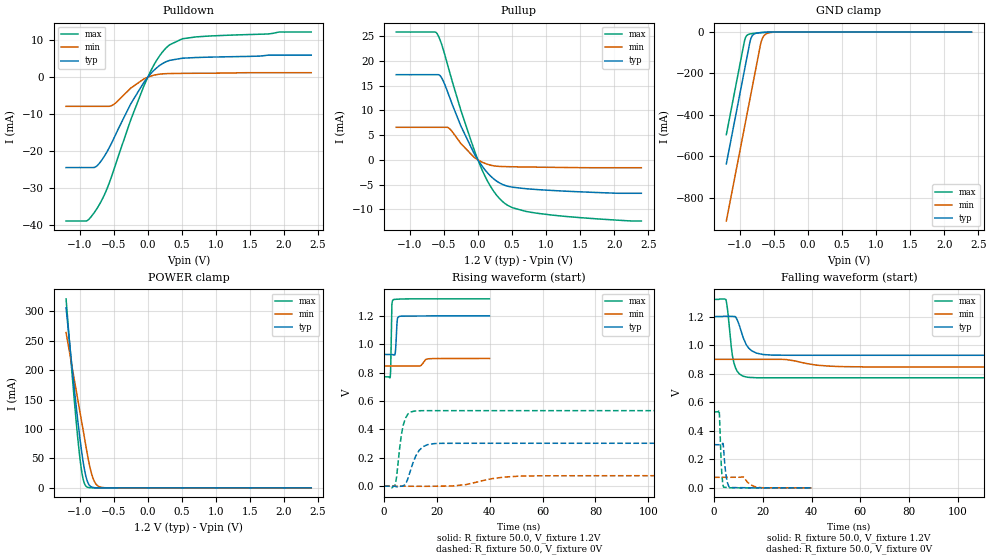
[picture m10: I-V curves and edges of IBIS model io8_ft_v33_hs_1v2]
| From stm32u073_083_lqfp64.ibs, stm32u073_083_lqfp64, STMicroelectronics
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[Model]   io8_ft_v33_hs_1v2
Model_type I/O
Polarity   Non-Inverting
Enable   Active-Low
| CAP_THRESHOLD on pad IOFT is "UDTCAPC" :
| Rising=30.0% of vddiom   Falling=70.0% of vddiom
| C_comp min and max val. don't necessarily correlate with the min and max pvt
| but are the smallest and greatest pad capacitance found.
| var   typ   min   max
C_comp   1.89804pF  1.82360pF  1.89870pF
|C_comp_pullup   1.10155pF  1.05685pF  1.08560pF
|C_comp_pulldown   796.48500fF  766.74501fF  813.10001fF
Vinl = 270.0mV
Vinh = 924.0mV
Vmeas = 600.0mV   | Reference voltage for timing measurements
Cref  = 50.0pF   | Timing specification test load capacitance value
Rref  = 100.0MOhm   | Timing specification test load resistance value
Vref  = 600.0mV   | Timing specification test load voltage
[Model Spec]
| TIME_THRESHOLD on pin ZIV33M is "CMOS" :
| Rising=50.0% of vddiom   Falling=50.0% of vddiom
Vinl 458.70000mV 364.70000mV 499.70000mV
Vinh 728.30000mV 548.30000mV 792.30000mV
| variable   typ   min   max
[Temperature Range] 25.0 140.0 -40.0
| variable   typ   min   max
[Voltage Range] 1.2V 900.0mV 1.32V
| variable   typ   min   max
[POWER Clamp Reference] 1.2V 900.0mV 1.32V
| variable   typ   min   max
[GND Clamp Reference] 0V 0V 0V
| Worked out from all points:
|   slope of the pulldown table from 0 to 0.18 V, typ, clamps not added: 55.6 ohm
|   slope of the pullup table from 0 to 0.18 V, typ, clamps not added: 56.3 ohm
|   GND clamp passes 1 mA (typ) near -0.61 V on its own axis
|   POWER clamp passes 1 mA (typ) near -0.81 V on its own axis
|   rising waveform, R_fixture 50.0, V_fixture 1.2V: 20-80 % time 435ps typ, 1.27ns min, 277ps max; typ from 0.928 V to 1.2 V
|   falling waveform, R_fixture 50.0, V_fixture 1.2V: 20-80 % time 3.79ns typ, 10.5ns min, 2.27ns max; typ from 1.2 V to 0.928 V
|   rising waveform, R_fixture 50.0, V_fixture 0V: 20-80 % time 3.76ns typ, 11.5ns min, 2.21ns max; typ from 0 V to 0.302 V
|   falling waveform, R_fixture 50.0, V_fixture 0V: 20-80 % time 1.14ns typ, 2.92ns min, 784ps max; typ from 0.302 V to 0 V
[POWER Clamp]
-1.2V     306.2mA    263.9mA    321.2mA
-1.09V    180mA      191mA      163.4mA
-1.05V    136.9mA    164.5mA    110.9mA
-1.01V    96.55mA    138mA      64.02mA
-960mV    52.29mA    104.9mA    20.68mA
-930mV    31.08mA    85.01mA    7.282mA
-900mV    15.67mA    65.13mA    2.025mA
-850mV    3.417mA    35.2mA     196.2uA
-800mV    570.2uA    14.97mA    18.13uA
-750mV    88.98uA    4.952mA    1.667uA
-680mV    6.495uA    823.9uA    58.96nA
2.4V      0A         0A         0A
[GND Clamp]
-1.2V     -636.9mA   -913.2mA   -495.8mA
-940mV    -194.9mA   -471.2mA   -53.78mA
-920mV    -160.9mA   -437.2mA   -28.06mA
-890mV    -109.9mA   -386.2mA   -14.28mA
-850mV    -43.09mA   -318.2mA   -9.18mA
-820mV    -18.33mA   -267.2mA   -7.516mA
-780mV    -7.695mA   -199.2mA   -5.87mA
-690mV    -2.548mA   -49.42mA   -2.9mA
-660mV    -1.868mA   -24.06mA   -2.112mA
-630mV    -1.326mA   -12.18mA   -1.447mA
-430mV    -19.32uA   -177.8uA   -8.091uA
2.4V      298.5pA    77.04nA    207.1pA
| variable   typ   min   max
[Pullup Reference] 1.2V 900.0mV 1.32V
| variable   typ   min   max
[Pulldown Reference] 0V 0V 0V
[Pullup]
-1.2V     17.25mA    6.594mA    25.88mA
-630mV    17.25mA    6.594mA    25.88mA
-600mV    17.25mA    6.594mA    25.56mA
-530mV    16.54mA    6.594mA    23.27mA
-420mV    12.82mA    6.361mA    17.99mA
-250mV    6.833mA    3.302mA    10.02mA
10mV      -217.3uA   -81.33uA   -351.4uA
200mV     -3.465mA   -1.119mA   -5.704mA
390mV     -5.137mA   -1.365mA   -8.762mA
510mV     -5.544mA   -1.401mA   -9.708mA
900mV     -6.043mA   -1.482mA   -10.87mA
2.4V      -6.768mA   -1.593mA   -12.38mA
[Pulldown]
-1.2V     -24.47mA   -7.9mA     -38.94mA
-890mV    -24.47mA   -7.9mA     -38.83mA
-720mV    -23.49mA   -7.9mA     -34.76mA
-610mV    -20.54mA   -7.9mA     -30.69mA
-510mV    -17.01mA   -7.49mA    -25.69mA
-250mV    -7.205mA   -2.955mA   -11.53mA
0V        -15fA      0A         0A
160mV     2.97mA     779.9uA    5.417mA
320mV     4.547mA    983.4uA    8.763mA
510mV     5.135mA    1.031mA    10.4mA
700mV     5.311mA    1.057mA    10.88mA
2.4V      5.965mA    1.209mA    12.22mA
[Ramp]
dV/dt_r 181.27275mV/3.7575ns 44.08574mV/11.4637ns 319.2097mV/2.20258ns
dV/dt_f 162.9125mV/3.78456ns 32.16353mV/10.51946ns 329.56981mV/2.27015ns
R_load = 50.0
| Removed startup time: 0s 0s 0s  .
| Removed end time: 39.9ns.
[Rising Waveform]
R_fixture   = 50.0
V_fixture   = 1.2V
V_fixture_min = 900.0mV
V_fixture_max = 1.32V
0s        928.4mV    846.4mV    770.7mV
2.4ns     928.5mV    846.4mV    772.7mV
2.6ns     928.6mV    846.4mV    868.6mV
2.9ns     928.5mV    846.4mV    1.223V
3ns       928.4mV    846.4mV    1.276V
3.5ns     926.5mV    846.4mV    1.314V
4.3ns     941.9mV    846.4mV    1.317V
5ns       1.165V     846.4mV    1.317V
5.7ns     1.195V     846.4mV    1.318V
39.9ns    1.2V       899.8mV    1.32V
| Removed startup time: 0s 0s 0s  .
| Removed end time: 149.9ns.
[Falling Waveform]
R_fixture   = 50.0
V_fixture   = 1.2V
V_fixture_min = 900.0mV
V_fixture_max = 1.32V
0s        1.2V       900mV      1.32V
4.9ns     1.202V     900mV      1.317V
5.7ns     1.202V     900mV      1.223V
6.9ns     1.202V     900mV      1.008V
8ns       1.201V     900mV      883.7mV
10.4ns    1.136V     900mV      797.1mV
13.8ns    987.7mV    900.6mV    774.1mV
23.4ns    929.9mV    900.3mV    770.7mV
51.9ns    928.4mV    849.2mV    770.7mV
149.9ns   928.5mV    846.4mV    770.7mV
| Removed startup time: 0s 0s 0s  .
| Removed end time: 149.9ns.
[Rising Waveform]
R_fixture   = 50.0
V_fixture   = 0V
V_fixture_min = 0V
V_fixture_max = 0V
0s        -2.581uV   2.34uV     -6.091uV
4.3ns     -1.839mV   -106.7nV   12.34mV
6.1ns     -1.067mV   -299.3nV   293.6mV
7.3ns     963.1uV    -669.7nV   430mV
9ns       49.85mV    1.138uV    506.8mV
11.4ns    183.4mV    32.1uV     529mV
14.7ns    277.2mV    -979.7uV   531.9mV
18.8ns    299.5mV    -389.9uV   532mV
51.1ns    302.1mV    70.28mV    532mV
149.9ns   302.1mV    73.48mV    532mV
| Removed startup time: 0s 0s 0s  .
| Removed end time: 39.9ns.
[Falling Waveform]
R_fixture   = 50.0
V_fixture   = 0V
V_fixture_min = 0V
V_fixture_max = 0V
0s        302.1mV    73.45mV    532mV
2.1ns     302mV      73.46mV    541.7mV
3ns       302.1mV    73.46mV    148.8mV
3.5ns     311.6mV    73.46mV    35.4mV
3.9ns     275.6mV    73.46mV    4.886mV
5ns       78.15mV    73.46mV    2.396mV
6.6ns     2.023mV    73.43mV    643.3uV
12ns      304.1uV    76.04mV    33.58uV
17.8ns    37.41uV    3.31mV     1.778uV
39.9ns    1.494uV    56.47uV    -2.785uV
